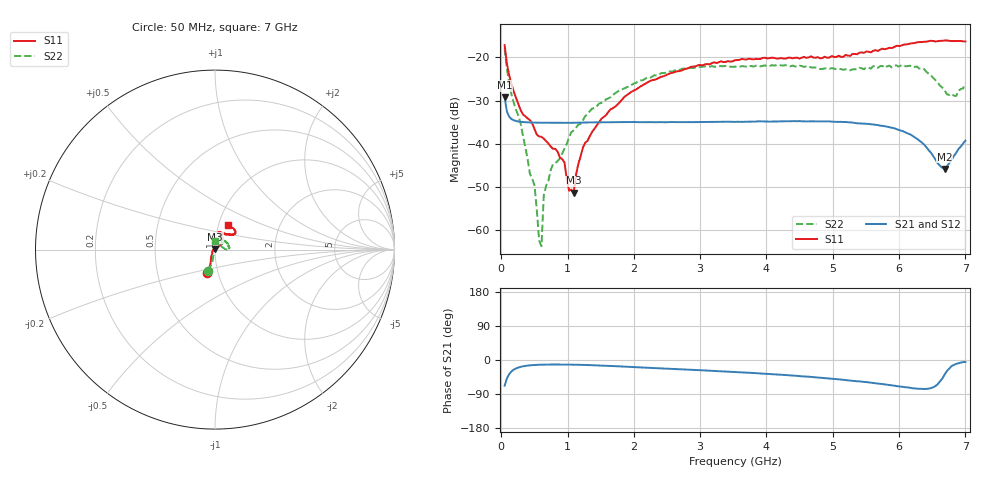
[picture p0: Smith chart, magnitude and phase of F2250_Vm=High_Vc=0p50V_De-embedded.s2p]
! Integrated Device Technology
! Corporate Headquarters
! 6024 Silver Creek Valley Road
! San Jose, CA 95138  USA
! Phone:  1-408-284-8200
! Toll Free:  1-800-223-1366
! Webpage:  http://www.idt.com/
! Timing and RF Division
! 515 Groton Road, Suite 102
! Westford, MA 01886-6024
! Device:  F2250
! Description: Voltage Variable RF Attenuator
! Frequency:  50.0 -  6000.00 MHz
! Package:  3x3 mm Thin QFN Plastic Package: 16 pin
! Ports:  2 RF, 3 DC
!  Pin  1  = GND
!  Pin  2  = NC
!  Pin  3  = RF1  = Port 1
!  Pin  4  = NC
!  Pin  5  = GND
!  Pin  6  = GND
!  Pin  7  = GND
!  Pin  8  = GND
!  Pin  9  = NC
!  Pin 10  = RF2  = Port 2
!  Pin 11  = NC
!  Pin 12  = GND
!  Pin 13  = GND
!  Pin 14  = VCNTRL
!  Pin 15  = VDD
!  Pin 16  = VMODE
! Vcntrl:  0.500 Volts
! Vmode:  +3.300 Volts
! Vdd:  +3.30  Volts
! Current:  1.267 mA
! Data:  The device was measured on a the F2250 evaluation board which has
!  individual transmission lines to the RF pins.  Data was collected
!  using a calibrated network analyzer.  The evaluation board was
!  de-embedded using a TRL calibration technique.
!  The reference plane is the edge of the package pin.
! Misc:  SN 10
!  Action Tracker AT0258
! Date Measured:  2014-11-26
! Date:  2015-10-15  MJV
! Note:
!  Integrated Device Technology supplies this data as a sample of measured
!  data at the package pin for this product.  Your particular data for this
!  product may vary.
!  Data was taken at 25 degrees C.
!  Integrated Device Technology reserves the right to change this data at anytime.
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# GHz S dB R 50
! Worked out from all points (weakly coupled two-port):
!   201 points, 50 MHz to 7 GHz, reference 50 ohm
!   highest |S21| = -29.22 dB at 50 MHz (marker M1); lowest = -45.8 dB at 6.687 GHz (marker M2)
!   lowest |S11| = -51.3 dB at 1.093 GHz (marker M3), VSWR 1.01, Z = 50 + j0.272 ohm
!   |S11| at or under -10 dB: start of sweep to end of sweep
!   |S22| runs from -63.7 to -18.0 dB; largest |S21 - S12| = 5.7e-05
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0.05  -17.17 -108.4  -29.22 -67.7  -29.22 -67.7  -17.95 -107.6
0.1195  -24.20 -111.9  -33.75 -37.1  -33.75 -37.1  -26.08 -103.1
0.29325  -32.28 -127.3  -34.92 -18.0  -34.92 -18.0  -35.41 -101.3
0.43225  -34.54 -145.1  -35.07 -14.1  -35.06 -14.1  -46.99 -115.1
0.50175  -36.63 -147.8  -35.10 -13.2  -35.10 -13.2  -49.69 -119.6
0.57125  -38.29 -161.0  -35.13 -12.6  -35.12 -12.6  -62.41 -146.0
0.606  -38.39 -162.5  -35.14 -12.4  -35.13 -12.4  -63.68 26.8
0.64075  -38.81 -162.3  -35.14 -12.2  -35.14 -12.2  -51.90 46.1
0.6755  -39.37 -163.8  -35.14 -12.1  -35.14 -12.1  -49.73 55.6
0.9535  -44.32 171.0  -35.16 -12.0  -35.17 -12.0  -41.12 56.5
1.023  -50.85 140.2  -35.15 -12.2  -35.15 -12.2  -38.44 47.5
1.0925  -51.32 87.8  -35.14 -12.4  -35.14 -12.3  -36.89 46.5
1.2315  -40.83 40.4  -35.09 -12.9  -35.10 -12.9  -34.55 36.0
1.6485  -32.01 41.1  -35.02 -15.7  -35.02 -15.7  -29.22 38.9
2.37825  -24.75 46.6  -34.99 -21.8  -34.99 -21.8  -24.03 42.6
3.525  -20.66 71.7  -34.93 -31.7  -34.93 -31.8  -22.15 66.7
4.7065  -20.06 72.0  -34.80 -45.2  -34.80 -45.2  -22.37 66.6
5.85325  -17.79 40.5  -36.18 -66.0  -36.18 -66.1  -21.92 17.4
6.3745  -16.40 40.9  -40.13 -76.6  -40.14 -76.6  -22.69 1.0
6.68725  -16.11 47.8  -45.80 -38.1  -45.79 -38.0  -27.62 23.1
6.861  -16.22 54.5  -42.09 -10.1  -42.06 -10.2  -28.93 58.8
7  -16.33 62.4  -39.26 -5.2  -39.23 -5.4  -26.02 88.9
